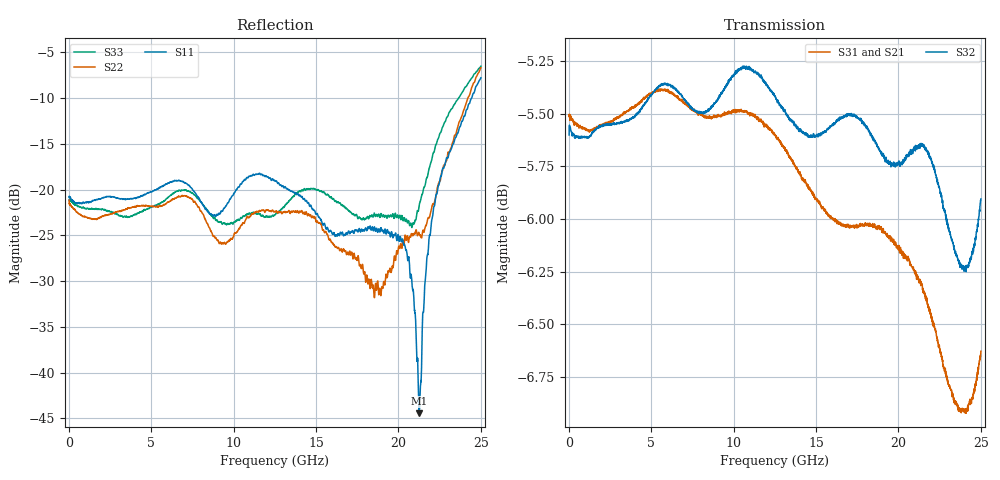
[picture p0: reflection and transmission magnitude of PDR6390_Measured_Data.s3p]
!The following data was pulled from an Agilent PNA
!This sNp file was generated from the data in the RF Test software
!NOTE:  Smoothing/Math/Corrections applied on any given trace ARE included in the data saved here
# MHz S dB R 50
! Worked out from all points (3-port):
!   2500 points, 10 MHz to 25 GHz, reference 50 ohm
!   strongest paths, dB at 10 MHz, 6.26 GHz, 12.51 GHz, 18.76 GHz, 25 GHz:
!     S32: -5.6, -5.4, -5.4, -5.7, -5.9
!     S31: -5.5, -5.4, -5.6, -6.0, -6.6
!     S21: -5.6, -5.5, -5.7, -6.2, -6.5
!   lowest |S11| = -44.5 dB at 21.25 GHz (marker M1), VSWR 1.01, Z = 50.2 + j0.564 ohm
!   |S11| at or under -10 dB: start of sweep to 24.44 GHz
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10  -20.82 -177.1  -5.61 0.5  -5.52 0.0
    -5.61 0.2  -21.17 -176.6  -5.64 0.1
    -5.51 0.0  -5.60 0.2  -21.20 -176.0
9350  -22.26 -168.5  -5.56 -22.3  -5.50 -23.9
      -5.56 -22.4  -25.92 -165.3  -5.39 -29.8
      -5.51 -23.9  -5.39 -29.8  -23.67 -157.7
12510  -19.08 -133.0  -5.68 -30.3  -5.60 -33.8
       -5.67 -30.3  -22.41 -143.3  -5.42 -42.3
       -5.60 -33.8  -5.42 -42.3  -22.76 -144.0
18560  -24.21 -107.5  -6.19 -44.1  -6.03 -48.7
       -6.18 -44.2  -31.51 -43.7  -5.63 -61.2
       -6.03 -48.8  -5.63 -61.1  -22.74 -66.6
20200  -25.61 -22.8  -6.20 -48.6  -6.15 -53.7
       -6.21 -48.6  -26.37 -35.0  -5.73 -65.8
       -6.17 -53.6  -5.73 -65.6  -22.83 -51.0
20860  -30.96 6.5  -6.25 -51.0  -6.23 -55.8
       -6.24 -51.1  -25.04 -46.7  -5.68 -68.0
       -6.23 -55.8  -5.69 -68.0  -23.76 -69.0
21250  -44.45 69.6  -6.32 -52.6  -6.29 -57.2
       -6.31 -52.7  -24.79 -58.6  -5.63 -69.7
       -6.30 -57.2  -5.65 -69.7  -21.84 -88.8
21690  -28.38 -163.9  -6.45 -54.3  -6.39 -59.0
       -6.45 -54.3  -23.89 -83.6  -5.67 -71.9
       -6.39 -59.0  -5.67 -71.9  -18.83 -100.1
22210  -21.57 -141.7  -6.66 -56.1  -6.51 -61.0
       -6.64 -56.2  -21.18 -100.4  -5.77 -74.5
       -6.52 -61.0  -5.77 -74.5  -15.50 -104.9
25000  -7.78 -32.4  -6.53 -61.4  -6.61 -67.5
       -6.50 -61.4  -6.69 -40.7  -5.89 -81.7
       -6.63 -67.5  -5.91 -81.7  -6.51 -41.0
